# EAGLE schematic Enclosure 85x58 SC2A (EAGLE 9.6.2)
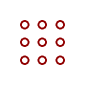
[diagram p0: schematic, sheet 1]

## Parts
U$1  PROTO-28X18-S2A  [PROTO-28X18-S2A]

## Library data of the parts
U$1 = digitalconcepts:PROTO-28X18-S2A: 28 x 18 Prototyping board to fit an 85 x 58 enclosure, with external connector cut-outs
